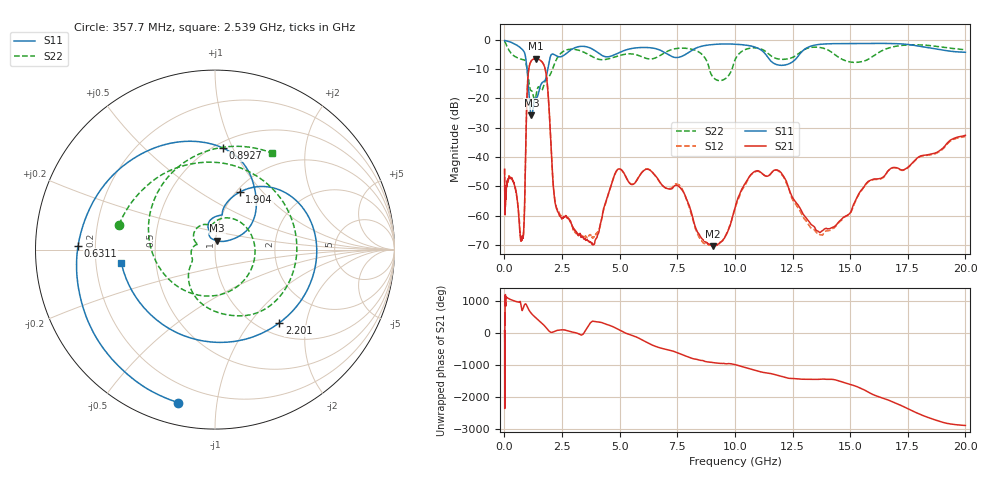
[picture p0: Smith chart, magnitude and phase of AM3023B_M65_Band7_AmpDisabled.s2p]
!Agilent Technologies,E8364B,MY43040894,A.07.50.67
!Agilent E8364B: A.07.50.67
!Date: Tuesday, October 27, 2020 10:49:58
!Correction: S11(Full 2 Port(1,2))
!S21(Full 2 Port(1,2))
!S12(Full 2 Port(1,2))
!S22(Full 2 Port(1,2))
!S2P File: Measurements: S11, S21, S12, S22:Log Frequency Sweep
# Hz S  dB  R 50
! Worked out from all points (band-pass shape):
!   3201 points, 10 MHz to 20 GHz, reference 50 ohm
!   highest |S21| = -6.51 dB at 1.362 GHz (marker M1); lowest = -70.4 dB at 9.047 GHz (marker M2)
!   |S21| within 3 dB of the highest: 1.069 GHz to 1.753 GHz (683.3 MHz wide, 48.4 % of centre)
!   lowest |S11| = -25.8 dB at 1.17 GHz (marker M3), VSWR 1.11, Z = 51 + j5.07 ohm
!   |S11| at or under -10 dB: 983.5 MHz to 1.884 GHz (900.7 MHz wide, 62.8 % of centre)
!   |S22| runs from -20.3 to -0.6 dB; largest |S21 - S12| = 0.0073
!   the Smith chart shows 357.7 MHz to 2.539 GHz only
!   S11 on the Smith chart (normalised r, x): 357.7 MHz: 0.11, -0.78; 631.1 MHz: 0.13, +0.01; 892.7 MHz: 0.55, +0.92; 1.904 GHz: 1.04, +0.76; 2.201 GHz: 1.22, -1.41; 2.539 GHz: 0.31, -0.06
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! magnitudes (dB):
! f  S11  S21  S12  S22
! 10 MHz  -0.3  -44.2  -44.0  -0.7
! 35.55 MHz  -0.4  -58.4  -56.4  -0.9
! 126.1 MHz  -0.5  -48.6  -48.5  -2.5
! 357.7 MHz  -1.1  -47.8  -47.9  -5.2
! 447.2 MHz  -1.5  -49.8  -49.5  -5.7
! 631.1 MHz  -2.4  -60.7  -59.8  -6.4
! 809.9 MHz  -3.6  -67.6  -67.0  -6.8
! 892.7 MHz  -4.9  -50.7  -51.3  -7.1
! 1.003 GHz  -11.7  -15.2  -15.2  -10.8
! 1.17 GHz  -25.8  -7.2  -7.2  -17.4
! 1.362 GHz  -19.9  -6.5  -6.5  -19.4
! 1.59 GHz  -15.3  -7.2  -7.3  -17.3
! 1.904 GHz  -9.1  -19.3  -19.3  -12.9
! 2.201 GHz  -5.3  -55.7  -55.1  -7.7
! 2.539 GHz  -5.6  -60.8  -60.5  -4.1
! 3.829 GHz  -3.3  -69.9  -67.6  -5.9
! 5.639 GHz  -2.9  -49.0  -49.0  -5.0
! 7.57 GHz  -6.0  -50.1  -49.4  -2.9
! 9.047 GHz  -1.7  -70.4  -69.7  -12.7
! 10.81 GHz  -2.4  -45.2  -45.3  -2.8
! 13.91 GHz  -1.5  -64.4  -65.5  -3.1
! 20 GHz  -4.3  -32.6  -33.0  -3.5
